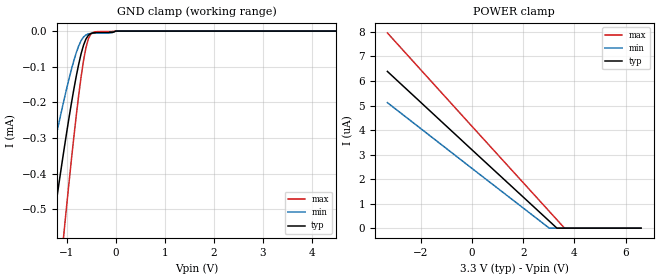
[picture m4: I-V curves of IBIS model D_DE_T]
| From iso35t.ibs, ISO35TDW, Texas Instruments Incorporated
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|   Driver Input/ Enable  for ISO35T
[Model]   D_DE_T
Model_type   Input
|Signals   DE/D
Vinl   = 0.99V
Vinh   = 2.31V
|   typ   min   max
|ccomp   (typ PVT)   (Slow PVT)   (Fast PVT)
C_comp   0.25330443pF   0.25330442pF   0.25330444pF
[Model Spec]
Vinl   0.99V   0.9V   1.08V
Vinh   2.31V   2.1V   2.52V
|   typ   min   max
[Temperature Range]   27.0   85   -40
[Voltage range]   3.3V   3.0V   3.6V
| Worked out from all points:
|   GND clamp passes 1 mA (typ) near -1.74 V on its own axis
[GND Clamp]
|   Voltage   I(typ)   I(min)   I(max)
-3.3V     -2.747mA   -1.859mA   -4.192mA
-1.609V   -863.1uA   -555.7uA   -1.366mA
-1.31V    -567.1uA   -351.9uA   -921.6uA
-1.26V    -518.9uA   -319uA     -849uA
-1.061V   -332.9uA   -193.4uA   -565uA
-912.1mV  -204.4uA   -108.9uA   -363.5uA
-762.8mV  -94.03uA   -42.17uA   -182uA
-663.3mV  -40.1uA    -16.82uA   -83.66uA
-563.8mV  -11.98uA   -7.942uA   -21.91uA
-464.3mV  -4.925uA   -6.144uA   -3.589uA
0V        0A         0A         0A
6.6V      0A         0A         0A
[POWER Clamp]
|   Voltage   I(typ)   I(min)   I(max)
-3.3V     6.39uA     5.118uA    7.961uA
3.018V    287.6nA    0A         685.8nA
3.317V    0A         0A         342.9nA
3.615V    0A         0A         0A
6.6V      0A         0A         0A
